FUNCTION "ASSE Y" : VOID
TITLE =GESTIONE SEGNALI DI STATO E COMANDO DELL'ASSE X
VERSION : 0.1

BEGIN
NETWORK
TITLE =INS./DISIN.1
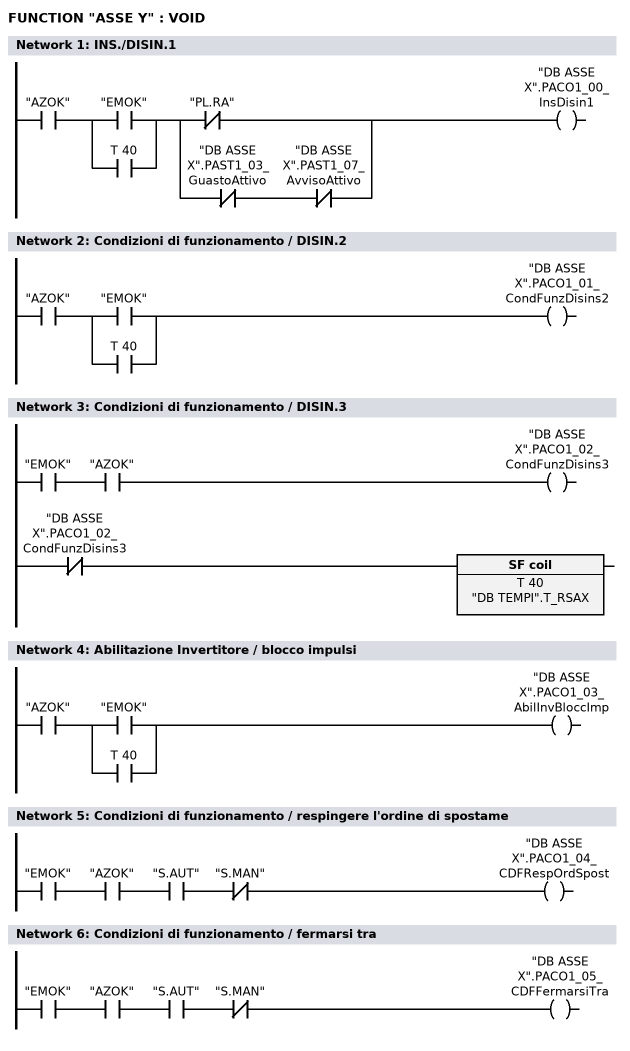
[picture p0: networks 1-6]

      U     "AZOK";
      U(    ;
      O     "EMOK";
      O     T     40;
      )     ;
      U(    ;
      UN    "PL.RA";
      O     ;
      UN    "DB ASSE X".PAST1_03_GuastoAttivo;
      UN    "DB ASSE X".PAST1_07_AvvisoAttivo;
      )     ;
      =     "DB ASSE X".PACO1_00_InsDisin1;

NETWORK
TITLE =Condizioni di funzionamento / DISIN.2

      U     "AZOK";
      U(    ;
      O     "EMOK";
      O     T     40;
      )     ;
      =     "DB ASSE X".PACO1_01_CondFunzDisins2;

NETWORK
TITLE =Condizioni di funzionamento / DISIN.3

      U     "EMOK";
      U     "AZOK";
      =     "DB ASSE X".PACO1_02_CondFunzDisins3;
//---------------------------
      UN    "DB ASSE X".PACO1_02_CondFunzDisins3;
      L     "DB TEMPI".T_RSAX;
      SA    T     40;

NETWORK
TITLE =Abilitazione Invertitore / blocco impulsi

      U     "AZOK";
      U(    ;
      O     "EMOK";
      O     T     40;
      )     ;
      =     "DB ASSE X".PACO1_03_AbilInvBloccImp;

NETWORK
TITLE =Condizioni di funzionamento / respingere l'ordine di spostame

      U     "EMOK";
      U     "AZOK";
      U     "S.AUT";
      UN    "S.MAN";
      =     "DB ASSE X".PACO1_04_CDFRespOrdSpost;

NETWORK
TITLE =Condizioni di funzionamento / fermarsi tra

      U     "EMOK";
      U     "AZOK";
      U     "S.AUT";
      UN    "S.MAN";
//      UN    M    125.6     ciclo sospeso
      =     "DB ASSE X".PACO1_05_CDFFermarsiTra;

NETWORK
TITLE =Attivare l'ordine di spostamento ( Fronte )

      CLR   ;
//      U     M    134.4    richiesta avvio blocco spost. da ciclo aut
      =     "DB ASSE X".PACO1_06_AttOverrSpostam;

NETWORK
TITLE =Reset memoria guasti
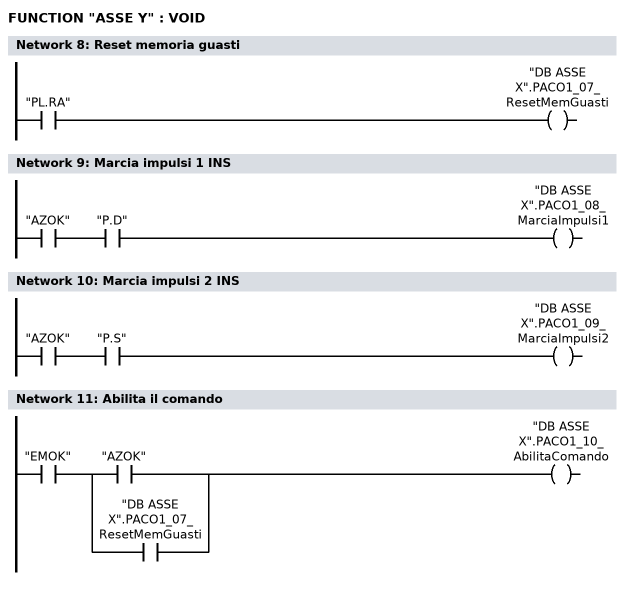
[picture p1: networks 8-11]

      U     "PL.RA";
      =     "DB ASSE X".PACO1_07_ResetMemGuasti;

NETWORK
TITLE =Marcia impulsi 1 INS

      U     "AZOK";
      U     "P.D";
      =     "DB ASSE X".PACO1_08_MarciaImpulsi1;

NETWORK
TITLE =Marcia impulsi 2 INS

      U     "AZOK";
      U     "P.S";
      =     "DB ASSE X".PACO1_09_MarciaImpulsi2;

NETWORK
TITLE =Abilita il comando

      U     "EMOK";
      U(    ;
      U     "AZOK";
      O     ;
      U     "DB ASSE X".PACO1_07_ResetMemGuasti;
      )     ;
      =     "DB ASSE X".PACO1_10_AbilitaComando;

NETWORK
TITLE =Avvio a riferirsi

      CLR   ;
      U     "EMOK";
      U     "AZOK";
//      U     M     32.4    azzeramento in corso
//      UN    M     32.6    asse x non sincronizzato
      =     "DB ASSE X".PACO1_11_AvvioRiferirsi;

NETWORK
TITLE =Cambio del blocco esterno

      CLR   ;
      =     "DB ASSE X".PACO1_13_CambioBloccoExt;

NETWORK
TITLE =Caricamento del numero blocco di spostamento desiderato



NETWORK
TITLE =Funzionamento a seguire

      CLR   ;
      =     "DB ASSE X".POSPACO_00_FunzASeguire;

NETWORK
TITLE =Imposta il punto di riferimento

      CLR   ;
      =     "DB ASSE X".POSPACO_01_ImpostPuntRif;

NETWORK
TITLE =Camma di riferimento

      UN    "FC.ZX";
      =     "DB ASSE X".POSPACO_02_CammaRiferime;

NETWORK
TITLE =Sensore della battuta fissa

      CLR   ;
      =     "DB ASSE X".POSPACO_03_SensBattFissa;

NETWORK
TITLE =Attivare l'accoppiamento

      CLR   ;
      =     "DB ASSE X".POSPACO_04_AttivAccoppia;

NETWORK
TITLE =Commutazione del blocco di parametri Bit 0

      CLR   ;
      =     "DB ASSE X".PACO2_00_CommBlocParBit1;

NETWORK
TITLE =Commutazione del blocco di parametri Bit 1

      CLR   ;
      =     "DB ASSE X".PACO2_01_CommBlocParBit2;

NETWORK
TITLE =Commutazione del blocco di parametri Bit 2

      CLR   ;
      =     "DB ASSE X".PACO2_02_CommBlocParBit3;

NETWORK
TITLE =Primo filtro nel riferimento di velocita' disinserito

      CLR   ;
      =     "DB ASSE X".PACO2_03_1FiltRifVelDisi;

NETWORK
TITLE =Tempo rampa zero

      CLR   ;
      =     "DB ASSE X".PACO2_04_TempoRampaZero;

NETWORK
TITLE =Blocco dell'integratore nel regolatore di velocita'

      CLR   ;
      =     "DB ASSE X".PACO2_06_BlocIntegrRegV;

NETWORK
TITLE =Scelta dell'asse in parcheggio

      CLR   ;
      =     "DB ASSE X".PACO2_07_SceltaAsseInPar;

NETWORK
TITLE =Tacitare il guasto 608

      U     "AZOK";
      U     "PL.RA";
      =     "DB ASSE X".PACO2_08_TacitGuasto608;

NETWORK
TITLE =Commutazione dati del motore 1 ingresso

      CLR   ;
      =     "DB ASSE X".PACO2_09_CommDatiMot1Ing;

NETWORK
TITLE =Commutazione dati del motore 2 ingresso

      CLR   ;
      =     "DB ASSE X".PACO2_10_CommDatiMot2Ing;

NETWORK
TITLE =Ha luogo la ommutazione del motore

      CLR   ;
      =     "DB ASSE X".PACO2_11_CommutazMotore;

NETWORK
TITLE =OVERRIDE

      U     "M.MAN";
      UN    "S.JV";
      SPBN  E001;
      L     DB102.DBW   20;
      T     "DB ASSE X".OVERRIDE;
      T     DB102.DBW   24;
E001: NOP   0;
      U     "M.AZZ";
      U     "S.JV";
      SPBN  E002;
      L     DB102.DBW   20;
      L     2;
      *I    ;
      T     "DB ASSE X".OVERRIDE;
      T     DB102.DBW   24;
E002: NOP   0;
      UN    "M.MAN";
      SPBN  E003;
      L     DB102.DBW   22;
      T     "DB ASSE X".OVERRIDE;
      T     DB102.DBW   24;
E003: NOP   0;

NETWORK
TITLE =Riduzione percentuale del limite di coppia

      L     0;
      T     "DB ASSE X".MOMRID;

NETWORK
TITLE =Caricamento quote

      SPA   fine;
      U     M     13.2;
      UN    M     14.0;
      S     M     14.0;
      S     M     14.1;
//============================ QUOTA 1
      U     M     14.1;
      SPBN  END1;
      L     W#16#8051;
      T     "DB ASSE X".PKE_Scrittura;
      L     W#16#1;
      T     "DB ASSE X".IND_Scrittura;
      L     DB104.DBD    2;
      T     DB121.DBD    4;
//----------------------------
      U(    ;
      L     "DB ASSE X".PKE_Lettura;
      L     W#16#5051;
      ==I   ;
      )     ;
      U(    ;
      L     "DB ASSE X".IND_Lettura;
      L     W#16#1;
      ==I   ;
      )     ;
      R     M     14.1;
      S     M     14.2;
END1: NOP   0;
//============================ QUOTA 2
      U     M     14.2;
      SPBN  END2;
      L     W#16#8051;
      T     "DB ASSE X".PKE_Scrittura;
      L     W#16#2;
      T     "DB ASSE X".IND_Scrittura;
      L     DB104.DBD   14;
      T     DB121.DBD    4;
//----------------------------
      U(    ;
      L     "DB ASSE X".PKE_Lettura;
      L     W#16#5051;
      ==I   ;
      )     ;
      U(    ;
      L     "DB ASSE X".IND_Lettura;
      L     W#16#2;
      ==I   ;
      )     ;
      R     M     14.2;
      S     M     14.3;
END2: NOP   0;
//============================ QUOTA 3
      U     M     14.3;
      SPBN  END3;
      L     W#16#8051;
      T     "DB ASSE X".PKE_Scrittura;
      L     W#16#3;
      T     "DB ASSE X".IND_Scrittura;
      L     DB104.DBD   26;
      T     DB121.DBD    4;
//----------------------------
      U(    ;
      L     "DB ASSE X".PKE_Lettura;
      L     W#16#5051;
      ==I   ;
      )     ;
      U(    ;
      L     "DB ASSE X".IND_Lettura;
      L     W#16#3;
      ==I   ;
      )     ;
      R     M     14.3;
      S     M     14.4;
END3: NOP   0;
//============================ VELOCITA' 1
      U     M     14.4;
      SPBN  END4;
      L     W#16#8052;
      T     "DB ASSE X".PKE_Scrittura;
      L     W#16#1;
      T     "DB ASSE X".IND_Scrittura;
      L     DB104.DBD   66;
      T     DB121.DBD    4;
//----------------------------
      U(    ;
      L     "DB ASSE X".PKE_Lettura;
      L     W#16#5052;
      ==I   ;
      )     ;
      U(    ;
      L     "DB ASSE X".IND_Lettura;
      L     W#16#1;
      ==I   ;
      )     ;
      R     M     14.4;
      S     M     14.5;
END4: NOP   0;
//============================ VELOCITA' 2
      U     M     14.5;
      SPBN  END5;
      L     W#16#8052;
      T     "DB ASSE X".PKE_Scrittura;
      L     W#16#2;
      T     "DB ASSE X".IND_Scrittura;
      L     DB104.DBD   66;
      T     DB121.DBD    4;
//----------------------------
      U(    ;
      L     "DB ASSE X".PKE_Lettura;
      L     W#16#5052;
      ==I   ;
      )     ;
      U(    ;
      L     "DB ASSE X".IND_Lettura;
      L     W#16#2;
      ==I   ;
      )     ;
      R     M     14.5;
      S     M     14.6;
END5: NOP   0;
//============================ VELOCITA' 3
      U     M     14.6;
      SPBN  END6;
      L     W#16#8052;
      T     "DB ASSE X".PKE_Scrittura;
      L     W#16#3;
      T     "DB ASSE X".IND_Scrittura;
      L     DB104.DBD   66;
      T     DB121.DBD    4;
//----------------------------
      U(    ;
      L     "DB ASSE X".PKE_Lettura;
      L     W#16#5052;
      ==I   ;
      )     ;
      U(    ;
      L     "DB ASSE X".IND_Lettura;
      L     W#16#3;
      ==I   ;
      )     ;
      R     M     14.6;
      S     M     14.7;
END6: NOP   0;
      U     M     14.7;
      UN    M     13.2;
      R     M     14.7;
      R     M     14.0;
fine: NOP   0;

NETWORK
TITLE =LETTURA ALLARMI

      U     "DB ASSE X".PAST1_03_GuastoAttivo;

END_FUNCTION

